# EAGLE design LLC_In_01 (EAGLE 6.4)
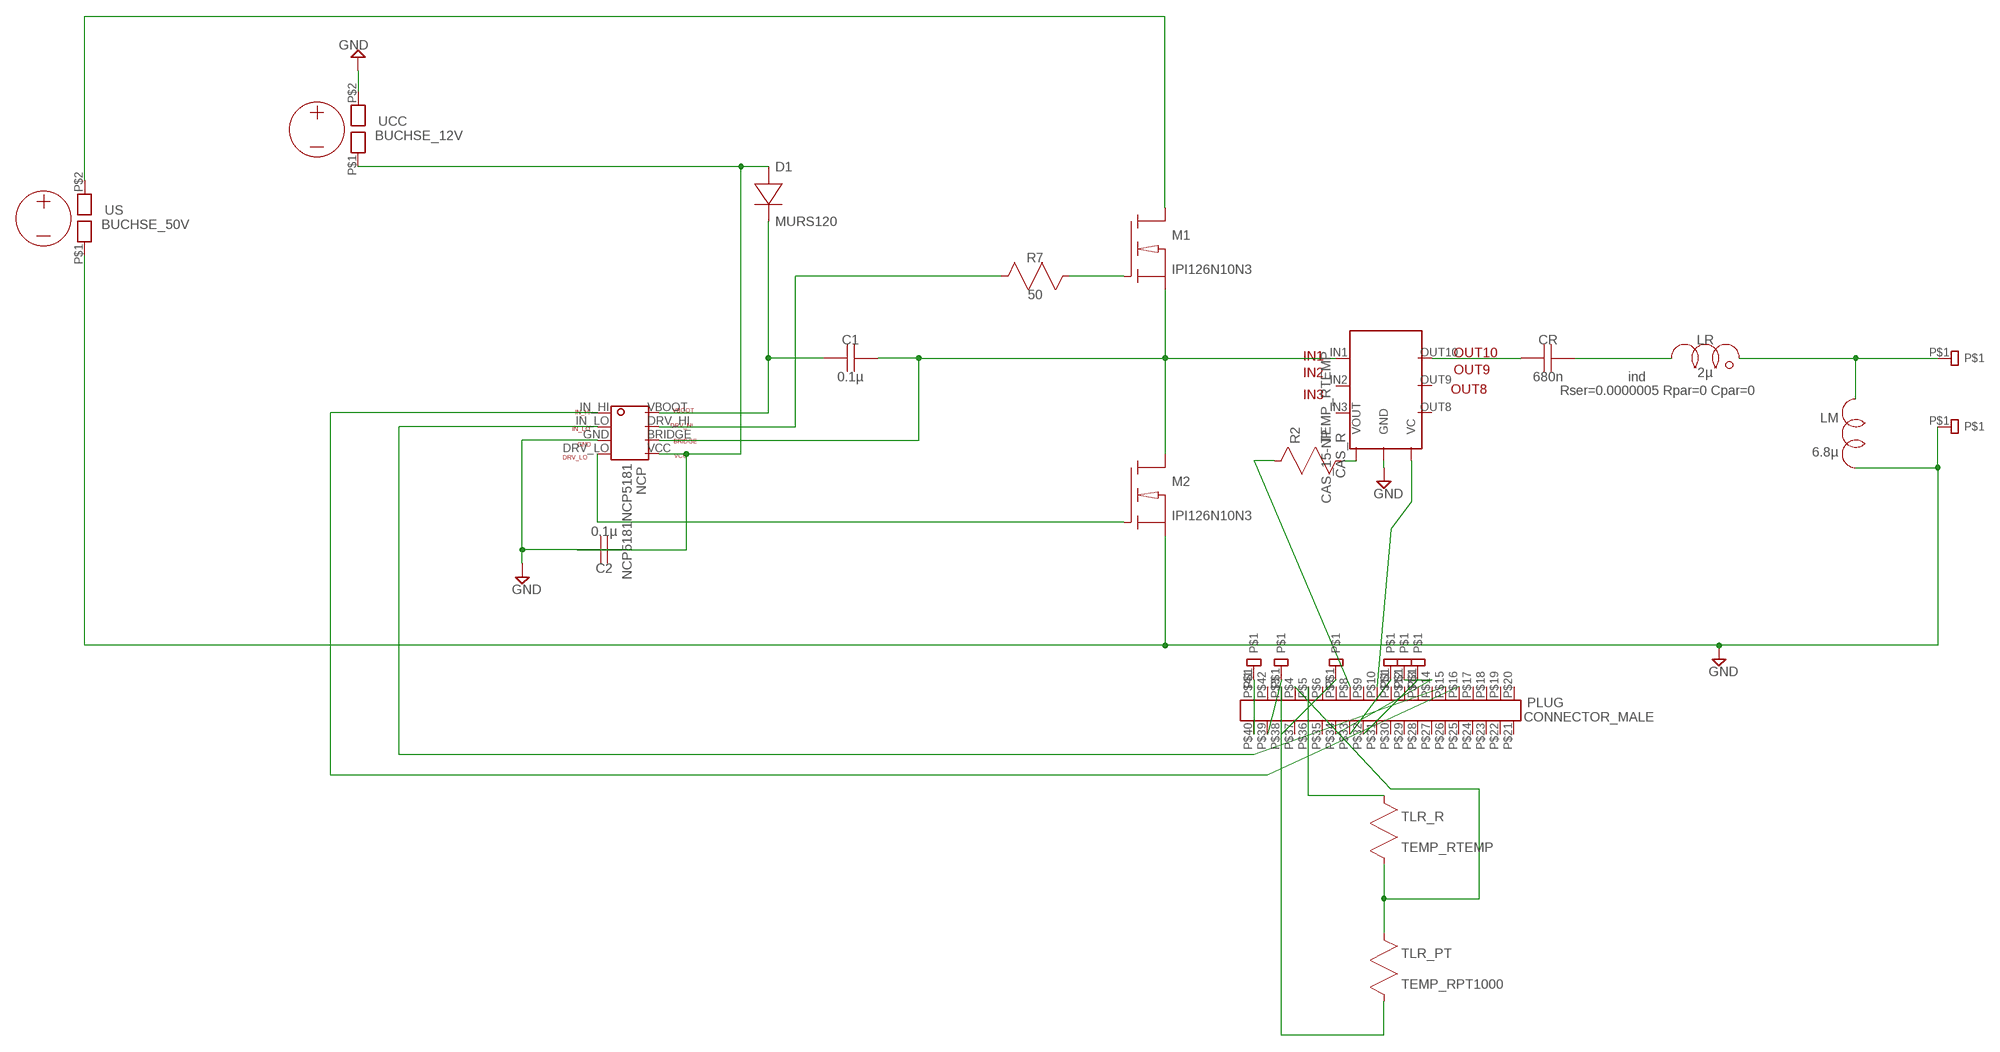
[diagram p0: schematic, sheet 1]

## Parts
C1  0.1µ  CAPC_BOOT_K  [C_BOOT_KER]
C2  0.1µ  CAPC_BOOT_K  [C_BOOT_KER]
CAS_R  CAS_15-NP  CAS_15-NPCAS_15-NP  [CAS_15-NP]
CR  680n  CAPCR  [CR_23MM_GRID]
D1  MURS120  DIODEDIODE_BOOT  [DIODE_BOOT]
LM  6.8µ  INDLM_NEU  [LM_NEU]
LR  2µ  IND2LR_SER2014  [LR_SER2014]
M1  IPI126N10N3  NMOSTO262-3-V  [T262-3-V]
M2  IPI126N10N3  NMOSTO262-3-V  [T262-3-V]
NCP  NCP5181NCP5181  [NCP5181]
PLUG  CONNECTOR_MALE  [CONNECTOR_MALE]
R2  TEMP_RTEMP  [TEMP_R]
R7  50  RESRES_MESS  [RES_PWR]
TLR_PT  TEMP_RPT1000  [PT1000]
TLR_R  TEMP_RTEMP  [TEMP_R]
TRAFO_+  B2BB2B  [B2B]
TRAFO_-  B2BB2B  [B2B]
TTR_GND  B2BB2B  [B2B]
TTR_V2  B2BB2B  [B2B]
TTR_VREF  B2BB2B  [B2B]
UCC  BUCHSE_12V  BUCHSE_50V50V  [BUCHSE_50V]
US  BUCHSE_50V  BUCHSE_50V50V  [BUCHSE_50V]
VCC_OUT  B2BB2B  [B2B]
VO  B2BB2B  [B2B]
VOUT_OUT  B2BB2B  [B2B]

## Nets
GND: C2.2(B) CAS_R.GND NCP.GND UCC.P$2
N$1: PLUG.P$5 TLR_R.1(A)
N$2: M1.1(G) R7.P$1(A)
N$3: M1.2(D) US.P$2
N$4: PLUG.P$3 TLR_PT.P$2(B)
N$5: NCP.DRV_HI R7.P$2(B)
N$6: PLUG.P$34 TTR_GND.P$1
N$7: CAS_R.OUT10 CR.1(A)
N$8: CR.2(B) LR.P$1(A)
N$9: LM.P$2(B) LR.P$2(B) TRAFO_+.P$1
N$10: LM.P$1(A) M2.3(S) TRAFO_-.P$1 US.P$1 ; supply symbol labelled GND
N$11: C1.2(B) D1.C(-) NCP.VBOOT
N$12: C1.1(A) CAS_R.IN1 M1.3(S) M2.2(D) NCP.BRIDGE
N$13: PLUG.P$8 R2.1(A)
N$14: CAS_R.VC PLUG.P$10
N$15: NCP.IN_HI PLUG.P$16
N$16: NCP.IN_LO PLUG.P$15
N$17: PLUG.P$33 TTR_VREF.P$1
N$18: PLUG.P$32 TTR_V2.P$1
N$19: M2.1(G) NCP.DRV_LO
N$20: CAS_R.VOUT R2.2(B)
N$21: PLUG.P$4 TLR_PT.P$1(A) TLR_R.2(B)
N$28: PLUG.P$40 VO.P$1
N$29: PLUG.P$39 VCC_OUT.P$1
N$31: PLUG.P$38 VOUT_OUT.P$1
VCC: C2.1(A) D1.A(+) NCP.VCC UCC.P$1
Unconnected: CAS_R.IN2 CAS_R.IN3 CAS_R.OUT8 CAS_R.OUT9 PLUG.P$6 PLUG.P$7 PLUG.P$9 PLUG.P$11 PLUG.P$12 PLUG.P$13 PLUG.P$14 PLUG.P$17 PLUG.P$18 PLUG.P$19 PLUG.P$20 PLUG.P$21 PLUG.P$22 PLUG.P$23 PLUG.P$24 PLUG.P$25 PLUG.P$26 PLUG.P$27 PLUG.P$28 PLUG.P$29 PLUG.P$30 PLUG.P$31 PLUG.P$35 PLUG.P$36 PLUG.P$37 PLUG.P$41 PLUG.P$42

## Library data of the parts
C1 C2 CR = sym:CAP: Capacitor
CAS_R = sym:CAS_15-NP
D1 = sym:DIODE: Diode
LM = sym:IND: Inductor; VALUE2: AC 50
LR = sym:IND2: Inductor; SPICELINE: Rser=0.0000005 Rpar=0 Cpar=0; SPICETYPE: ind
M1 M2 = sym:NMOS: N-Channel MOSFET transistor
NCP = sym:NCP5181
PLUG = sym:CONNECTOR_MALE
R2 TLR_PT TLR_R = sym:TEMP_R
R7 = sym:RES: A resistor
TRAFO_+ TRAFO_- TTR_GND TTR_V2 TTR_VREF VCC_OUT VO VOUT_OUT = sym:B2B
UCC US = sym:BUCHSE_50V

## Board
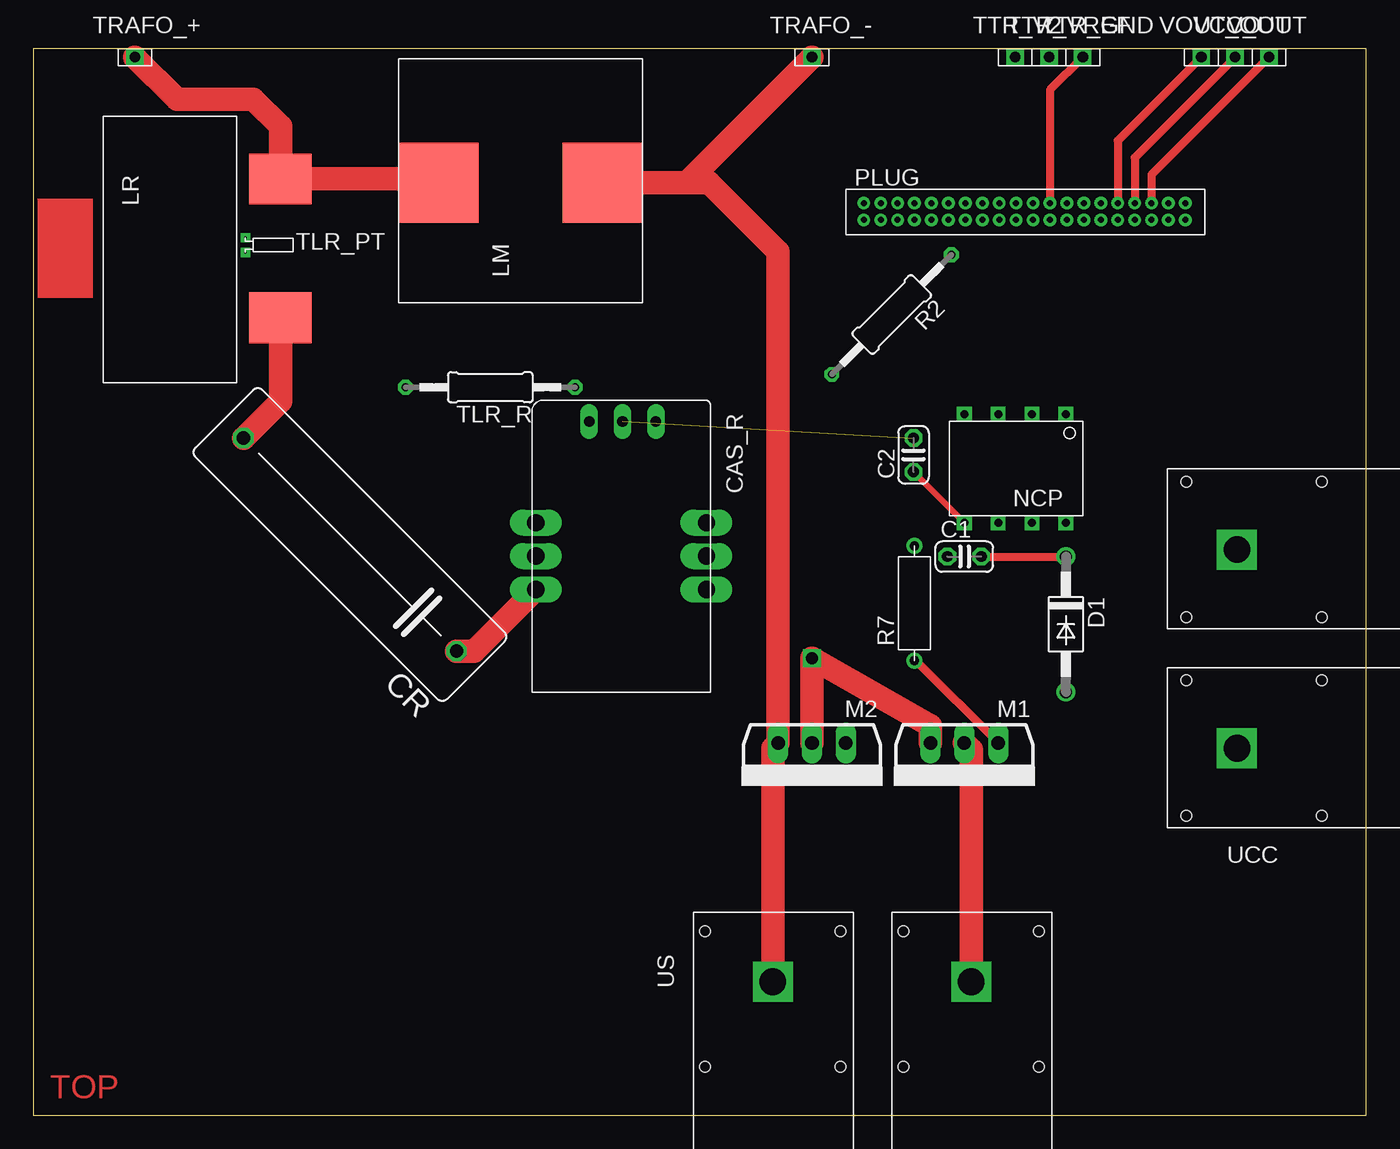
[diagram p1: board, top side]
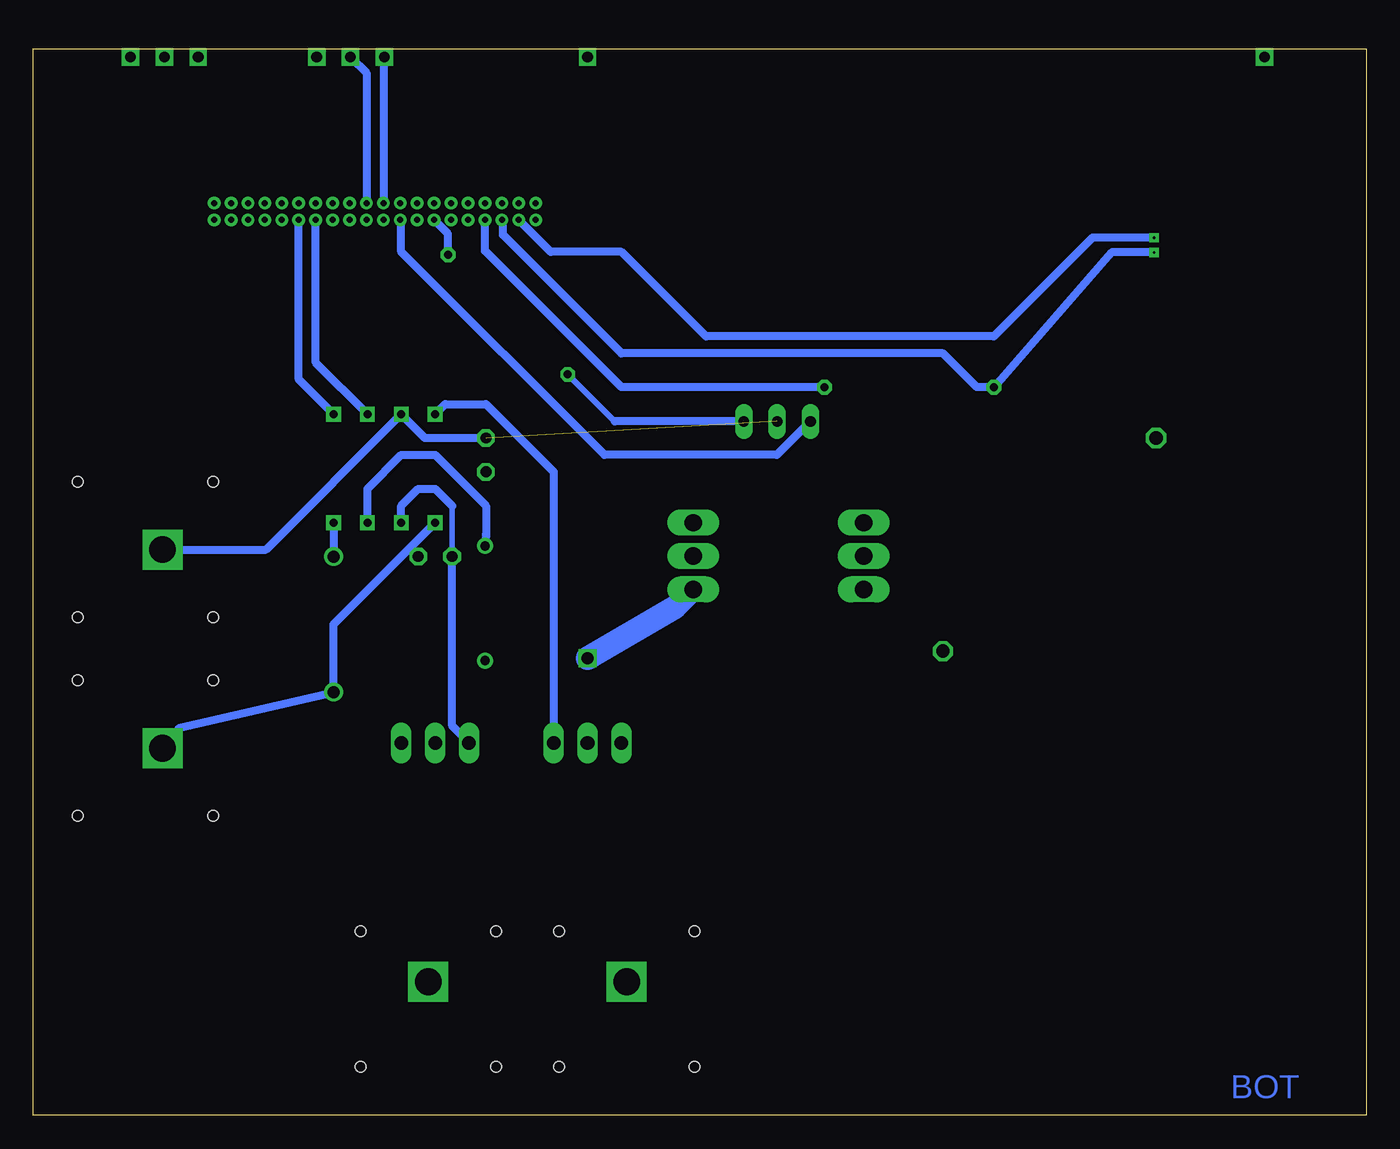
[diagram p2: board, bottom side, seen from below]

Size 100 x 80 mm. Coordinates in mm from the lower left corner, seen from the top.
Outline: 0,0 100,0 100,80 0,80 0,0
Copper layers (1*16): Top 0.035mm / dielectric 1.5mm / Bottom 0.035mm
Design rules "default *": minimum track width 10mil, minimum drill 0.15mm, track to track 8mil, track to pad 8mil, pad to pad 8mil, via to via 8mil, smd to smd 8mil, copper to edge 40mil, drill to drill 8mil, minimum pad ring 10mil, minimum via ring 8mil, stop-mask expansion 4mil, vias tented up to drill 0mil, thermal gap 10mil

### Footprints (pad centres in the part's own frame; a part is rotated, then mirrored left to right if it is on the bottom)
C_BOOT_KER = drill 0.813 octagon: 1 1.27,2.54; 2 3.81,2.54
CAS_15-NP = drill 0.8 pad 1.27 long: GND -10.14,-0.25; VC -10.14,-2.75; VOUT -10.14,2.25 | drill 1.3 long: IN1 2.46,6.05; IN2 -0.04,6.05; IN3 -2.54,6.05 | drill 1.3 pad 1.93 long: OUT8 -2.54,-6.75; OUT9 -0.04,-6.75; OUT10 2.46,-6.75
CR_23MM_GRID = drill 1 octagon: 1 -11.303,-1.27; 2 11.303,-1.27
DIODE_BOOT = drill 0.9: A 5.08,0; C -5.08,0
LM_NEU = smd 6 x 6: P$1 9,3; P$2 9,15.3
LR_SER2014 = smd 3.81 x 4.7: P$1 -15.1,-3.3; P$2 -4.7,-3.3
T262-3-V = drill 1.016 long: 1 -2.54,0; 2 0,0; 3 2.54,0
NCP5181 = drill 0.6 square: BRIDGE 6.35,7.62; DRV_HI 3.81,7.62; DRV_LO 8.89,-0.508; GND 6.35,-0.508; IN_HI 1.27,-0.508; IN_LO 3.81,-0.508; VBOOT 1.27,7.62; VCC 8.89,7.62
CONNECTOR_MALE = drill 0.45: P$1 1.346,1.118; P$2 1.346,1.118; P$3 2.616,1.118; P$4 3.886,1.118; P$5 5.156,1.118; P$6 6.426,1.118; P$7 7.696,1.118; P$8 8.966,1.118; P$9 10.236,1.118; P$10 11.506,1.118; P$11 12.776,1.118; P$12 14.046,1.118; P$13 15.316,1.118; P$14 16.586,1.118; P$15 17.856,1.118; P$16 19.126,1.118; P$17 20.396,1.118; P$18 21.666,1.118; P$19 22.936,1.118; P$20 24.206,1.118; P$21 25.476,1.118; P$22 1.346,2.388; P$23 1.346,2.388; P$24 2.616,2.388; P$25 3.886,2.388; P$26 5.156,2.388; P$27 6.426,2.388; P$28 7.696,2.388; P$29 8.966,2.388; P$30 10.236,2.388; P$31 11.506,2.388; P$32 12.776,2.388; P$33 14.046,2.388; P$34 15.316,2.388; P$35 16.586,2.388; P$36 17.856,2.388; P$37 19.126,2.388; P$38 20.396,2.388; P$39 21.666,2.388; P$40 22.936,2.388; P$41 24.206,2.388; P$42 25.476,2.388
TEMP_R = drill 0.6 octagon: 1 -6.35,1.27; 2 6.35,1.27
RES_PWR = drill 0.7: P$1 -7.8,1.2; P$2 0.8,1.2
PT1000 = drill 0.2 pad 0.254 square: P$1 -0.6,-0.054; P$2 -0.6,1.054
B2B = drill 0.8 square: P$1 1.27,0.635
BUCHSE_50V = drill 2 square: P$1 5.22,5.95; P$2 5.22,20.84 | hole 0.8: 1.42,0.87; 1.42,11.03; 11.58,0.87; 11.58,11.03; 1.42,15.76; 1.42,25.92; 11.58,15.76; 11.58,25.92

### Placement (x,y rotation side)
C1  67.31,39.37 0 top
C2  68.58,46.99 90 top
CAS_R  44.45,41.91 270 top
CR  22.86,41.91 135 top
D1  77.47,36.83 270 top
LM  45.72,60.96 90 top
LR  15.24,74.93 90 top
M1  69.85,27.94 180 top
M2  58.42,27.94 180 top
NCP  78.74,52.07 180 top
PLUG  60.96,66.04 0 top
R2  63.5,60.96 225 top
R7  67.31,41.91 90 top
TLR_PT  16.51,64.77 0 top
TLR_R  34.29,55.88 180 top
TRAFO_+  6.35,78.74 0 top
TRAFO_-  57.15,78.74 0 top
TTR_GND  77.47,78.74 0 top
TTR_V2  72.39,78.74 0 top
TTR_VREF  74.93,78.74 0 top
UCC  85.09,21.59 0 top
US  49.53,15.24 270 top
VCC_OUT  88.9,78.74 0 top
VO  91.44,78.74 0 top
VOUT_OUT  86.36,78.74 0 top

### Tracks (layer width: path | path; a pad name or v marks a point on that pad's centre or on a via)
GND  (1 unrouted)
  Bottom 0.61: UCC.P$2 82.54,42.43 NCP.GND 70.61,50.8 C2.2
N$1
  Bottom 0.61: TLR_R.1 55.88,54.61 66.12,64.85 PLUG.P$5
N$2
  Top 0.406: 66.22,34.11 R7.P$1
  Top 0.61: M1.1 66.22,34.11
N$3
  Top 1.778: US.P$2 70.37,27.42 M1.2
N$4
  Bottom 0.61: TLR_PT.P$2 20.54,65.82 27.94,58.42 49.53,58.42 55.88,64.77 61.19,64.77 PLUG.P$3
N$5
  Bottom 0.61: NCP.DRV_HI 74.93,46.99 72.39,49.53 69.85,49.53 66.04,45.72 66.04,43.58 R7.P$2
N$6
  Top 0.61: TTR_GND.P$1 76.28,76.91 PLUG.P$34
N$7
  Top 1.778: CAS_R.OUT10 33.07,34.82 CR.1
N$8
  Top 1.778: CR.2 18.54,53.58 LR.P$1
N$9
  Top 1.778: TRAFO_+.P$1 10.79,76.2 16.51,76.2 18.54,74.17 LR.P$2 30.15,70.23 LM.P$2
N$10
  Top 1.778: US.P$1 55.48,27.54 M2.3 55.88,64.77 50.69,69.96 49.01,69.96 | LM.P$1 48.26,69.96 49.01,69.96 | 49.01,69.96 TRAFO_-.P$1
N$11
  Top 0.61: C1.2 D1.C
  Bottom 0.61: NCP.VBOOT D1.C
N$12  (via drill 0.9)
  Top 1.778: M1.3 67.31,29.21 v58.42,34.29 M2.2
  Bottom 0.406: 68.58,45.72 C1.1
  Bottom 0.61: NCP.BRIDGE 72.39,45.72 71.12,46.99 69.85,46.99 68.58,45.72 | M1.3 68.58,29.21 C1.1
  Bottom 1.778: v58.42,34.29 51.85,38.1 CAS_R.IN1
N$13
  Bottom 0.61: R2.1 68.89,66.12 PLUG.P$8
N$14
  Bottom 0.406: 72.39,67.08 PLUG.P$10
  Bottom 0.61: CAS_R.VC 44.22,49.53 57.15,49.53 72.39,64.77 72.39,67.08
N$15
  Bottom 0.61: NCP.IN_HI 80.09,55.19 PLUG.P$16
N$16
  Bottom 0.61: NCP.IN_LO 78.82,56.46 PLUG.P$15
N$17
  Bottom 0.61: TTR_VREF.P$1 75.01,78.18 PLUG.P$33
N$18
  Bottom 0.406: TTR_V2.P$1 73.74,79.3
  Bottom 0.61: 73.74,79.3 PLUG.P$32
N$19
  Bottom 0.61: NCP.DRV_LO 69.09,53.34 66.04,53.34 60.96,48.26 M2.1
N$20
  Bottom 0.406: 56.39,52.05 R2.2
  Bottom 0.61: CAS_R.VOUT 56.39,52.05
N$21
  Bottom 0.61: TLR_PT.P$1 19.1,64.72 TLR_R.2 29.21,54.61 31.75,57.15 55.88,57.15 64.77,66.04 64.77,67.08 PLUG.P$4
N$28
  Top 0.61: VO.P$1 83.9,70.56 PLUG.P$40
N$29
  Top 0.61: VCC_OUT.P$1 82.63,71.83 PLUG.P$39
N$31
  Top 0.61: VOUT_OUT.P$1 81.36,73.1 PLUG.P$38
VCC
  Top 0.406: NCP.VCC C2.1
  Bottom 0.61: UCC.P$1 89.04,29.07 D1.A 77.47,36.83 NCP.VCC

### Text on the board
Top: TOP
Bottom: BOT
